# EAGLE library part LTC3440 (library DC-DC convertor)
LTC3440 DC-DC converter UP and Down DC-DC converter. Producted by LINEAR TECHNOLOGY.Co
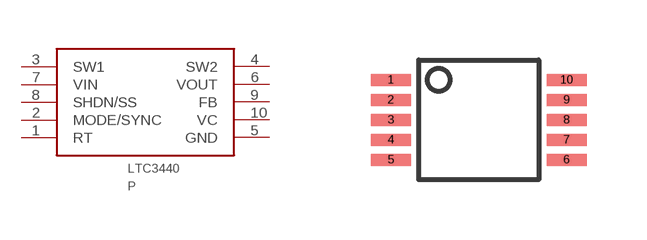
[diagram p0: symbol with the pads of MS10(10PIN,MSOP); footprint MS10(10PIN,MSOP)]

Designator prefix P

## LTC3440  [MS10(10PIN,MSOP)]
1  RT
2  MODE/SYNC
3  SW1
4  SW2
5  GND
6  VOUT
7  VIN
8  SHDN/SS
9  FB
10  VC

## Footprint MS10(10PIN,MSOP) (pad centres in mm)
MS10 package ; MSOP 10Pin (0.5pitch)
smd 1 x 0.3: 1 -2.2,1; 2 -2.2,0.5; 3 -2.2,0; 4 -2.2,-0.5; 5 -2.2,-1; 6 2.2,-1; 7 2.2,-0.5; 8 2.2,0; 9 2.2,0.5; 10 2.2,1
